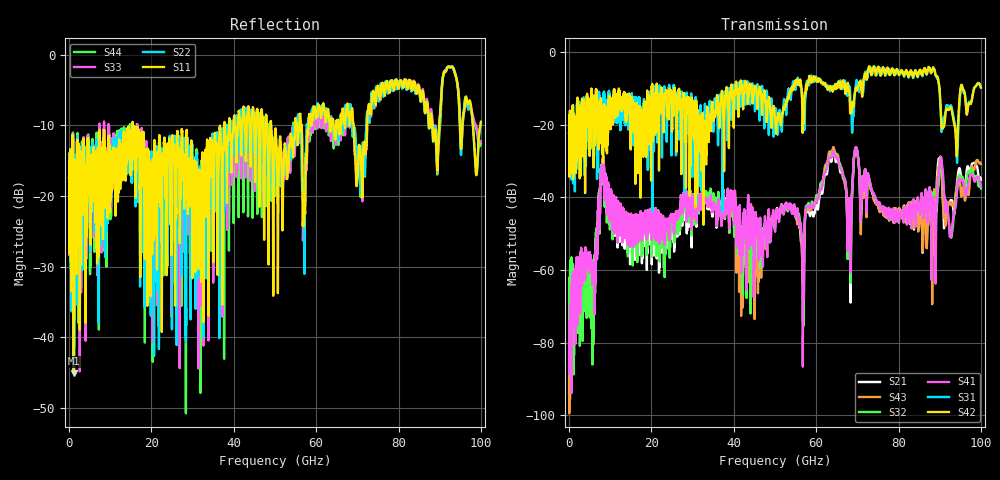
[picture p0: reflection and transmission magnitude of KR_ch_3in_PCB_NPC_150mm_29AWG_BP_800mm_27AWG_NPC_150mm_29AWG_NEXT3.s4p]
# GHz S RI R 45
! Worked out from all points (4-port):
!   4000 points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, 25 MHz to 100 GHz, reference 45 ohm
!   strongest paths, dB at 25 MHz, 25.02 GHz, 50.02 GHz, 75.03 GHz, 100 GHz:
!     S42: -22.2, -20.8, -18.7, -4.1, -9.8
!     S31: -22.2, -13.2, -15.7, -5.0, -9.6
!     S41: -86.4, -45.4, -49.4, -41.4, -37.0
!     S32: -84.0, -48.4, -47.2, -41.4, -37.5
!     S43: -88.5, -47.6, -46.3, -42.3, -30.8
!     S21: -94.1, -49.9, -47.3, -42.2, -35.2
!   lowest |S11| = -45.1 dB at 1.15 GHz (marker M1), VSWR 1.01, Z = 45.4 + j0.277 ohm
!   |S11| at or under -10 dB: start of sweep to 15.35 GHz; 15.47 GHz to 37.72 GHz (22.25 GHz wide, 83.7 % of centre); 49.09 GHz to 54.89 GHz (5.799 GHz wide, 11.2 % of centre)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
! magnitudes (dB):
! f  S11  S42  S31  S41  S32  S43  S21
! 25 MHz  -17.4  -22.2  -22.2  -86.4  -84.0  -88.5  -94.1
! 1.15 GHz  -45.1  -24.7  -27.3  -72.9  -88.7  -73.2  -75.1
! 5.85 GHz  -16.3  -11.9  -15.3  -60.2  -68.2  -73.1  -76.4
! 8.1 GHz  -15.1  -19.0  -23.6  -35.0  -34.8  -35.2  -34.8
! 56.67 GHz  -17.3  -19.8  -13.7  -56.8  -56.4  -60.5  -59.1
! 63.88 GHz  -9.3  -10.0  -9.5  -28.3  -28.3  -27.3  -29.0
! 100 GHz  -9.5  -9.8  -9.6  -37.0  -37.5  -30.8  -35.2
